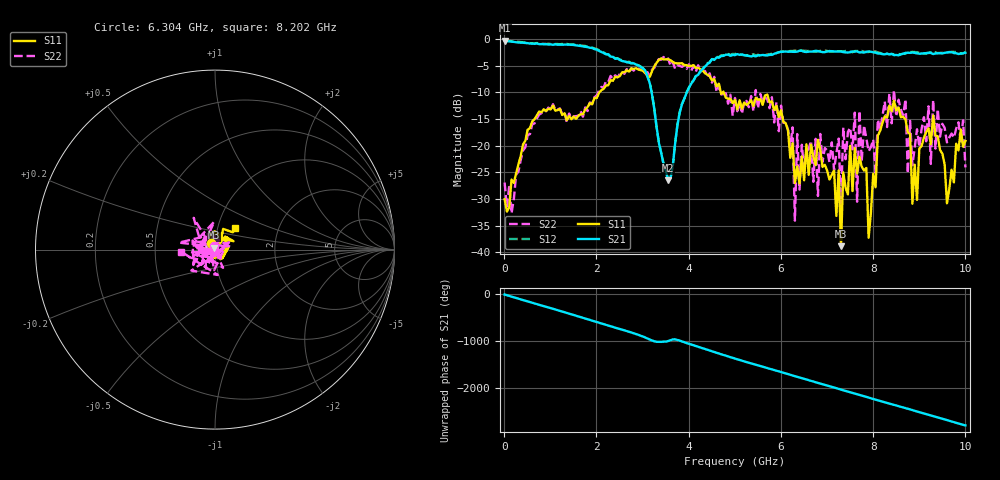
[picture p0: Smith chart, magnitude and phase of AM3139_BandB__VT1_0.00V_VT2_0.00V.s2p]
! Date/Time: Tue, Nov 13, 2018 4:59 PM
! Network Analyzer: Agilent Technologies E8364B Rev: A.07.50.67
! Sweep from 0.010 to 10.000 GHz, 201 Points, Sweep Type: LIN
! Power Supply: -0.000 V, 0.000 A
# Hz S DB R 50
!freq MagS11 AngS11 MagS21 AngS21 MagS12 AngS12 MagS22 AngS22
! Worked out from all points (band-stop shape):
!   201 points, 10 MHz to 10 GHz, reference 50 ohm
!   highest |S21| = -0.27 dB at 10 MHz (marker M1); lowest = -26.5 dB at 3.556 GHz (marker M2)
!   |S21| within 3 dB of the highest: start of sweep to 2.306 GHz; 4.689 GHz to end of sweep
!   lowest |S11| = -38.9 dB at 7.303 GHz (marker M3), VSWR 1.02, Z = 49.6 + j1.07 ohm
!   |S11| at or under -10 dB: start of sweep to 2.064 GHz; 4.698 GHz to 4.738 GHz (40.15 MHz wide, 0.851 % of centre); 4.762 GHz to end of sweep
!   |S22| runs from -34.1 to -3.3 dB; largest |S21 - S12| = 0.033
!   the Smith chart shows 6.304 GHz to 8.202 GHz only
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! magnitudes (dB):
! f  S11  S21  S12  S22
! 10 MHz  -30.1  -0.3  -0.2  -26.9
! 1.708 GHz  -14.1  -1.3  -1.2  -14.6
! 3.357 GHz  -3.9  -19.6  -19.5  -3.7
! 3.556 GHz  -3.7  -26.5  -26.5  -3.6
! 5.005 GHz  -11.4  -3.0  -2.8  -11.0
! 6.254 GHz  -19.6  -2.4  -2.2  -16.6
! 6.304 GHz  -27.0  -2.4  -2.1  -34.1
! 6.703 GHz  -22.0  -2.3  -2.3  -26.8
! 7.253 GHz  -24.7  -2.3  -2.3  -18.7
! 7.303 GHz  -38.9  -2.3  -2.2  -31.3
! 7.353 GHz  -25.0  -2.4  -2.3  -16.6
! 7.502 GHz  -20.0  -2.4  -2.3  -16.6
! 7.602 GHz  -20.4  -2.3  -2.2  -13.8
! 7.652 GHz  -25.2  -2.3  -2.2  -30.5
! 7.702 GHz  -22.1  -2.5  -2.3  -13.4
! 7.902 GHz  -37.3  -2.3  -2.4  -21.1
! 8.352 GHz  -12.5  -2.8  -2.8  -10.2
! 8.801 GHz  -17.8  -2.6  -2.4  -15.3
! 8.851 GHz  -30.9  -2.5  -2.4  -23.7
! 9.301 GHz  -14.3  -2.8  -2.6  -11.4
! 9.6 GHz  -30.8  -2.5  -2.4  -19.4
! 10 GHz  -19.1  -2.5  -2.5  -24.1
